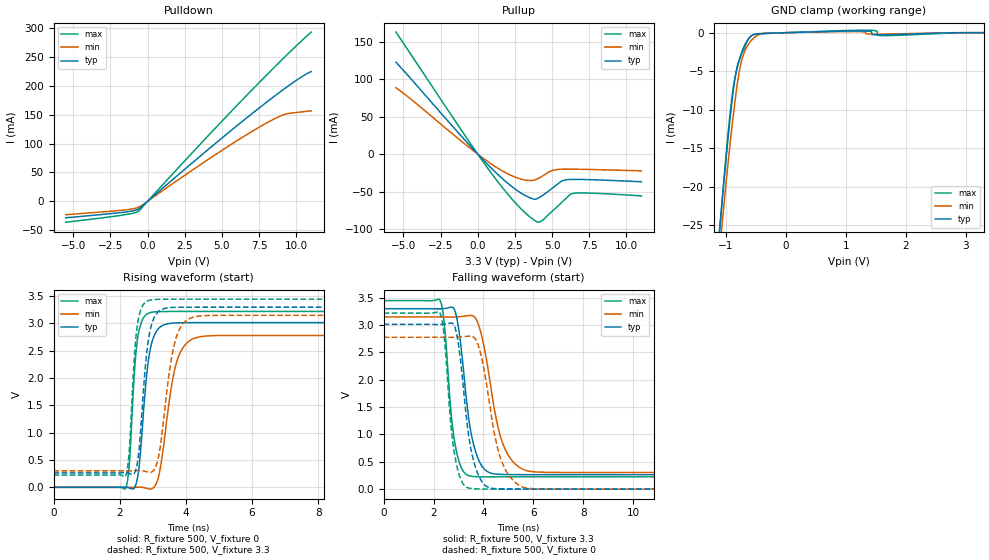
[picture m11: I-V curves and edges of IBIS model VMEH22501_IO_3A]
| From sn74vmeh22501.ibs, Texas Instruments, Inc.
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[Model]   VMEH22501_IO_3A
Model_type  I/O
Vinh =   2.0
Vinl =   0.8
Enable   Active-Low
Vref =   0
Rref =   500
Cref =   50p
Vmeas =   1.5
| variable   typ   min   max
C_comp   3.80pF   3.13pF   4.51pF
| C_pullup   3.10pF   2.08pF   4.55pF
| C_pulldown   2.52pF   1.95pF   3.11pF
| C_tri-state   3.80pF   3.13pF   4.51pF
[Temperature Range]   40   100   0
| Ambient temperature   25   85   0
[Voltage range]   3.3   3.15   3.45
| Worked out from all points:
|   slope of the pulldown table from 0 to 0.495 V, typ, clamps not added: 44.2 ohm
|   slope of the pullup table from 0 to 0.495 V, typ, clamps not added: 47.8 ohm
|   GND clamp passes 1 mA (typ) near -0.64 V on its own axis
|   rising waveform, R_fixture 500, V_fixture 0: 20-80 % time 269ps typ, 410ps min, 195ps max; typ from 0.001 V to 3.02 V
|   falling waveform, R_fixture 500, V_fixture 3.3: 20-80 % time 497ps typ, 709ps min, 370ps max; typ from 3.3 V to 0.265 V
|   rising waveform, R_fixture 500, V_fixture 3.3: 20-80 % time 254ps typ, 383ps min, 189ps max; typ from 0.265 V to 3.3 V
|   falling waveform, R_fixture 500, V_fixture 0: 20-80 % time 492ps typ, 685ps min, 371ps max; typ from 3.01 V to 0.001 V
[GND Clamp]
| VMEH22501_IO_3A
|   Voltage   I(typ)   I(min)   I(max)
-5.5V     -459.5mA   -438.5mA   -491.3mA
-1.105V   -25.79mA   -28.48mA   -25.96mA
-1.08V    -23.59mA   -26.39mA   -23.61mA
-1.055V   -21.42mA   -24.34mA   -21.29mA
-940mV    -12.02mA   -15.3mA    -11.41mA
-885mV    -8.156mA   -11.44mA   -7.694mA
-840mV    -5.648mA   -8.533mA   -5.594mA
-775mV    -3.529mA   -5.062mA   -3.617mA
-710mV    -2.05mA    -2.954mA   -2.311mA
-610mV    -684.7uA   -1.381mA   -693.1uA
-480mV    -146.4uA   -375.3uA   -172.7uA
3.3V      108pA      4.608nA    -720.6pA
[Pulldown]
| VMEH22501_IO_3A
|   Voltage   I(typ)   I(min)   I(max)
-5.5V     -28.59mA   -23.27mA   -36.27mA
-1.635V   -19.08mA   -15.31mA   -23.78mA
-905mV    -16.16mA   -12.58mA   -20.27mA
-600mV    -13.19mA   -10.16mA   -16.81mA
4.645V    102.1mA    82.34mA    129.3mA
6.435V    139.9mA    111.9mA    177.7mA
7.895V    169.7mA    134.3mA    216.1mA
8.73V     186.2mA    145.5mA    237.7mA
9.305V    197.2mA    151.4mA    252.4mA
10.34V    215.5mA    155mA      277.8mA
11V       224.9mA    156.9mA    293.4mA
[Pullup]
| VMEH22501_IO_3A
|   Voltage   I(typ)   I(min)   I(max)
-5.5V     122.7mA    88.67mA    162.8mA
-960mV    20.9mA     15.05mA    27.94mA
1.005V    -20.53mA   -14.36mA   -27.75mA
2.64V     -48.35mA   -31.65mA   -67.32mA
3.285V    -56.16mA   -34.82mA   -79.95mA
3.83V     -60.17mA   -34.4mA    -88.47mA
4.06V     -58.62mA   -32.42mA   -90.76mA
4.315V    -55.68mA   -29.67mA   -88.82mA
4.965V    -46.2mA    -22.17mA   -77mA
5.645V    -35.95mA   -20.12mA   -64.41mA
6.415V    -33.68mA   -20.06mA   -52.34mA
11V       -36.8mA    -22.29mA   -55.73mA
[Ramp]
| VMEH22501_IO_3A
| variable   typ   min   max
dV/dt_r   1.83/2.78E-10   1.69/4.23E-10   1.95/2.00E-10
dV/dt_f   1.84/5.04E-10   1.73/7.25E-10   1.95/3.74E-10
R_load = 500
[Rising Waveform]
| VMEH22501_IO_3A
R_fixture =   500
C_fixture =   0
L_fixture =   0
V_fixture =   0
V_fixture_min = 0
V_fixture_max = 0
|   Time   V(typ)   V(min)   V(max)
0s        754.1uV    2.345uV    2.693mV
2.185ns   4.451mV    -91.38uV   -12.54mV
2.29ns    -10.21mV   -230.2uV   418.7mV
2.54ns    180.9mV    3.755mV    2.721V
2.81ns    2.024V     -16.2mV    3.165V
2.965ns   2.638V     -26.12mV   3.204V
3.205ns   2.926V     279.6mV    3.217V
3.73ns    3.011V     2.311V     3.22V
4.38ns    3.015V     2.751V     3.22V
24.99ns   3.015V     2.78V      3.22V
[Falling Waveform]
| VMEH22501_IO_3A
R_fixture =   500
C_fixture =   0
L_fixture =   0
V_fixture =   3.3
V_fixture_min = 3.15
V_fixture_max = 3.45
|   Time   V(typ)   V(min)   V(max)
0s        3.299V     3.15V      3.447V
2.265ns   3.296V     3.15V      3.446V
2.425ns   3.303V     3.149V     3.043V
2.7ns     3.327V     3.147V     1.404V
2.895ns   3.2V       3.149V     742.5mV
3.43ns    1.228V     3.176V     244.7mV
3.9ns     450.4mV    2.856V     225.9mV
4.755ns   269.3mV    857.7mV    225.5mV
5.695ns   265.2mV    342.8mV    225.6mV
24.99ns   265.1mV    303.6mV    225.6mV
[Rising Waveform]
| VMEH22501_IO_3A
R_fixture =   500
C_fixture =   0
L_fixture =   0
V_fixture =   3.3
V_fixture_min = 3.15
V_fixture_max = 3.45
|   Time   V(typ)   V(min)   V(max)
0s        265.1mV    303.6mV    225.8mV
2.185ns   268.8mV    303.5mV    212.8mV
2.29ns    253.8mV    303.4mV    678.4mV
2.525ns   421.8mV    307.1mV    2.93V
2.795ns   2.339V     289mV      3.395V
2.93ns    2.903V     273.3mV    3.428V
3.18ns    3.221V     572mV      3.441V
3.69ns    3.295V     2.705V     3.443V
4.265ns   3.298V     3.122V     3.444V
24.99ns   3.299V     3.15V      3.446V
[Falling Waveform]
| VMEH22501_IO_3A
R_fixture =   500
C_fixture =   0
L_fixture =   0
V_fixture =   0
V_fixture_min = 0
V_fixture_max = 0
|   Time   V(typ)   V(min)   V(max)
0s        3.014V     2.778V     3.22V
2.26ns    3.012V     2.778V     3.218V
2.42ns    3.019V     2.777V     2.819V
2.69ns    3.036V     2.776V     1.199V
2.89ns    2.909V     2.78V      521.7mV
3.405ns   987.1mV    2.796V     21.28mV
3.865ns   194.8mV    2.517V     2.954mV
4.71ns    4.352mV    533.2mV    2.294mV
5.615ns   727.6uV    31.11mV    2.523mV
24.99ns   704.3uV    5.059uV    2.526mV
